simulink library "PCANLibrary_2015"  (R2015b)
settings: Solver=VariableStepAuto  SolverMode=SingleTasking  StartTime=0.0  StopTime=10.0  RelTol=1e-3
undefined symbols (not defined in the file or in its folder): FromID, hex2dec, Initvar, MsgFormat, PCAN_USBBUS, pcanchannel, ToID

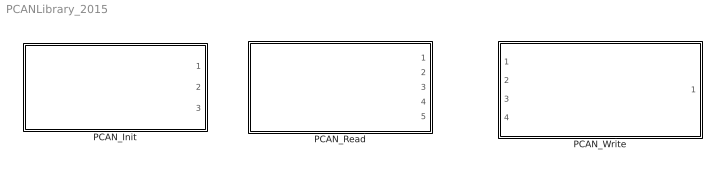
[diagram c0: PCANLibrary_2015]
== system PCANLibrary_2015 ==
  PCAN_Init : Subsystem
  PCAN_Read : Subsystem
  PCAN_Write : Subsystem

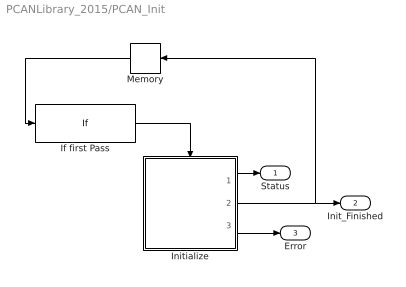
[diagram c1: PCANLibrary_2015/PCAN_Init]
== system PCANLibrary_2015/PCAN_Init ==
  If first Pass : If  IfExpression=u1 == 0  ShowElse=off
  Initialize : Subsystem  TreatAsAtomicUnit=on
  Memory : Memory  InheritSampleTime=on
  Status : Outport
  Init_Finished : Outport  Port=2
  Error : Outport  Port=3
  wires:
  If first Pass/1 -> Initialize/Action
  Initialize/1(Status) -> Status/1
  Memory/1 -> If first Pass/1
  Initialize/2(Init_Finished) -> Init_Finished/1, Memory/1
  Initialize/3(Error) -> Error/1

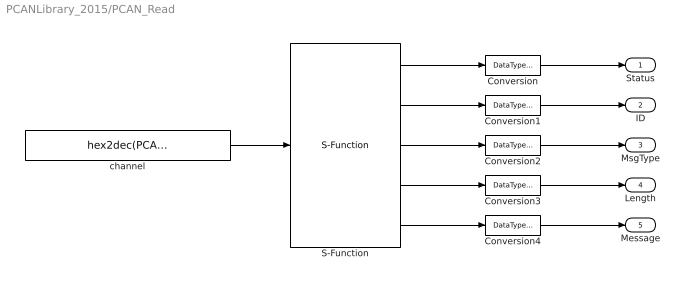
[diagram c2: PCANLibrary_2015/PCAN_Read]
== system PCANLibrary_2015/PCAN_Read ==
  Conversion : DataTypeConversion  OutDataTypeStr=uint32
  Conversion1 : DataTypeConversion  OutDataTypeStr=uint32
  Conversion2 : DataTypeConversion  OutDataTypeStr=uint8
  Conversion3 : DataTypeConversion  OutDataTypeStr=uint8
  Conversion4 : DataTypeConversion  OutDataTypeStr=uint8
  S-Function : S-Function  FunctionName=PCAN_Read  SFunctionDeploymentMode=off  EnableBusSupport=off
  channel : Constant  Value=hex2dec(PCAN_USBBUS)
  Status : Outport
  ID : Outport  Port=2
  MsgType : Outport  Port=3
  Length : Outport  Port=4
  Message : Outport  Port=5
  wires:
  S-Function/1 -> Conversion/1
  S-Function/2 -> Conversion1/1
  S-Function/3 -> Conversion2/1
  S-Function/4 -> Conversion3/1
  S-Function/5 -> Conversion4/1
  Conversion/1 -> Status/1
  Conversion1/1 -> ID/1
  Conversion2/1 -> MsgType/1
  Conversion3/1 -> Length/1
  Conversion4/1 -> Message/1
  channel/1 -> S-Function/1

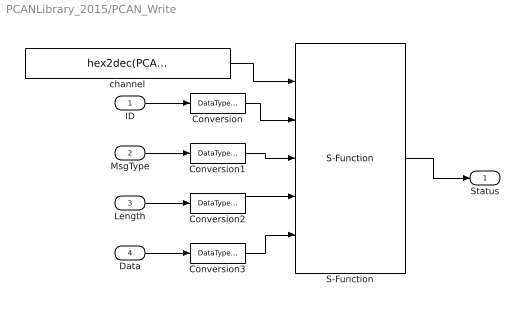
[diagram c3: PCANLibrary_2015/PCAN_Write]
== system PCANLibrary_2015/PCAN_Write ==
  ID : Inport  OutDataTypeStr=uint32
  MsgType : Inport  Port=2  OutDataTypeStr=uint8
  Length : Inport  Port=3  OutDataTypeStr=uint8
  Data : Inport  Port=4  OutDataTypeStr=uint8
  Conversion{,1..3} (4 alike) : DataTypeConversion  OutDataTypeStr=double
  S-Function : S-Function  FunctionName=PCAN_Write  SFunctionDeploymentMode=off  EnableBusSupport=off
  channel : Constant  Value=hex2dec(PCAN_USBBUS)
  Status : Outport
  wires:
  S-Function/1 -> Status/1
  ID/1 -> Conversion/1
  MsgType/1 -> Conversion1/1
  Length/1 -> Conversion2/1
  Data/1 -> Conversion3/1
  channel/1 -> S-Function/1
  Conversion/1 -> S-Function/2
  Conversion1/1 -> S-Function/3
  Conversion2/1 -> S-Function/4
  Conversion3/1 -> S-Function/5

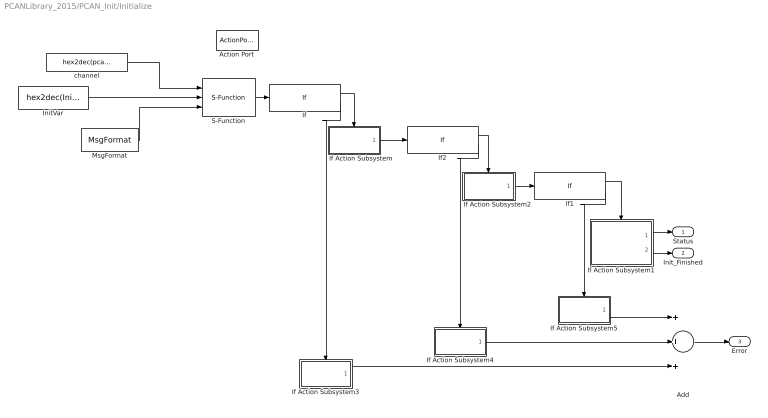
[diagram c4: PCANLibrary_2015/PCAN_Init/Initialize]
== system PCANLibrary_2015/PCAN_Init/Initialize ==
  Action Port : ActionPort
  Add : Sum  Inputs=+++
  If : If  IfExpression=u1== 0
  If Action Subsystem : Subsystem  TreatAsAtomicUnit=on
  If Action Subsystem1 : Subsystem  TreatAsAtomicUnit=on
  If Action Subsystem2 : Subsystem  TreatAsAtomicUnit=on
  If Action Subsystem3 : Subsystem  TreatAsAtomicUnit=on
  If Action Subsystem4 : Subsystem  TreatAsAtomicUnit=on
  If Action Subsystem5 : Subsystem  TreatAsAtomicUnit=on
  If1 : If  IfExpression=u1== 0
  If2 : If  IfExpression=u1== 0
  InitVar : Constant  Value=hex2dec(Initvar)
  MsgFormat : Constant  Value=MsgFormat
  S-Function : S-Function  FunctionName=PCAN_Init  SFunctionDeploymentMode=off  EnableBusSupport=off
  channel : Constant  Value=hex2dec(pcanchannel)
  Status : Outport  InitialOutput=0
  Init_Finished : Outport  Port=2  InitialOutput=0
  Error : Outport  Port=3  InitialOutput=0
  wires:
  S-Function/1 -> If/1
  If/1 -> If Action Subsystem/Action
  If Action Subsystem/1(Return) -> If2/1
  If Action Subsystem1/1(Status) -> Status/1
  If Action Subsystem1/2(Init_finish) -> Init_Finished/1
  If1/1 -> If Action Subsystem1/Action
  If2/1 -> If Action Subsystem2/Action
  If Action Subsystem2/1(return) -> If1/1
  If/2 -> If Action Subsystem3/Action
  If2/2 -> If Action Subsystem4/Action
  If1/2 -> If Action Subsystem5/Action
  If Action Subsystem5/1(Error) -> Add/1
  If Action Subsystem4/1(Error) -> Add/2
  If Action Subsystem3/1(Error) -> Add/3
  Add/1 -> Error/1
  MsgFormat/1 -> S-Function/3
  InitVar/1 -> S-Function/2
  channel/1 -> S-Function/1

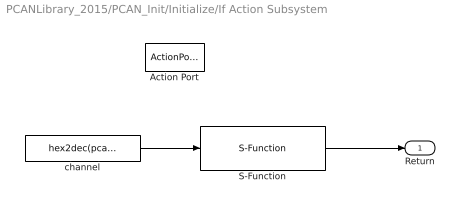
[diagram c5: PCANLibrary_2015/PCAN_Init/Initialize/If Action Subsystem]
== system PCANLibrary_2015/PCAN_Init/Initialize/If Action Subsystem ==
  Action Port : ActionPort
  S-Function : S-Function  FunctionName=PCAN_ResetFilter  SFunctionDeploymentMode=off  EnableBusSupport=off
  channel : Constant  Value=hex2dec(pcanchannel)
  Return : Outport
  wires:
  S-Function/1 -> Return/1
  channel/1 -> S-Function/1

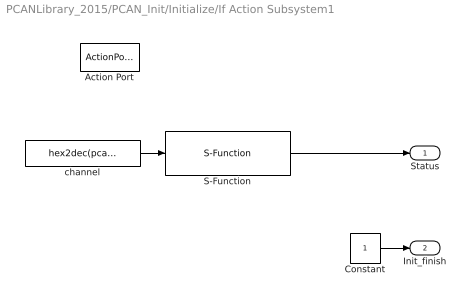
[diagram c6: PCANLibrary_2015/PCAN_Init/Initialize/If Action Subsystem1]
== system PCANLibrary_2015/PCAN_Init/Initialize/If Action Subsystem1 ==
  Action Port : ActionPort
  Constant : Constant
  S-Function : S-Function  FunctionName=PCAN_Status  SFunctionDeploymentMode=off  EnableBusSupport=off
  channel : Constant  Value=hex2dec(pcanchannel)
  Status : Outport
  Init_finish : Outport  Port=2
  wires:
  S-Function/1 -> Status/1
  Constant/1 -> Init_finish/1
  channel/1 -> S-Function/1

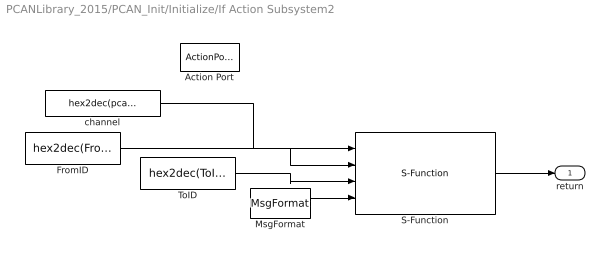
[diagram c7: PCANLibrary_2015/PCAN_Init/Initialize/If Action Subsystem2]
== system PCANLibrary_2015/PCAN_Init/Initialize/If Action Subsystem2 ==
  Action Port : ActionPort
  FromID : Constant  Value=hex2dec(FromID)
  MsgFormat : Constant  Value=MsgFormat
  S-Function : S-Function  FunctionName=PCAN_MsgFilter  SFunctionDeploymentMode=off  EnableBusSupport=off
  ToID : Constant  Value=hex2dec(ToID)
  channel : Constant  Value=hex2dec(pcanchannel)
  return : Outport
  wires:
  S-Function/1 -> return/1
  MsgFormat/1 -> S-Function/4
  ToID/1 -> S-Function/3
  FromID/1 -> S-Function/2
  channel/1 -> S-Function/1

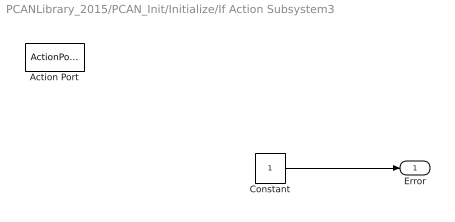
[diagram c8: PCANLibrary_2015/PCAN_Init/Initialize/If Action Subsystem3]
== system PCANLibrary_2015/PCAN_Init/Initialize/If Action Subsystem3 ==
  Action Port : ActionPort
  Constant : Constant
  Error : Outport  InitialOutput=0
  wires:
  Constant/1 -> Error/1

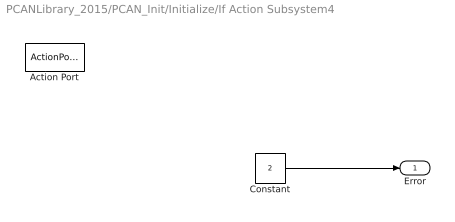
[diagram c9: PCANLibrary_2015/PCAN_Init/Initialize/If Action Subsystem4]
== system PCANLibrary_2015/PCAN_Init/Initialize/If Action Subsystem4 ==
  Action Port : ActionPort
  Constant : Constant  Value=2
  Error : Outport  InitialOutput=0
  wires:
  Constant/1 -> Error/1

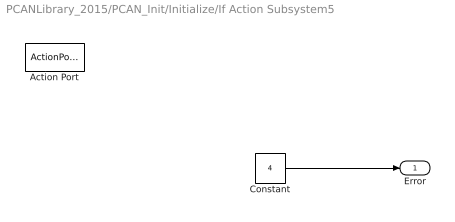
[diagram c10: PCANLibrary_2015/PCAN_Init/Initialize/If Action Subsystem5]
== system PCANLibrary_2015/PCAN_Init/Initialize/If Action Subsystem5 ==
  Action Port : ActionPort
  Constant : Constant  Value=4
  Error : Outport  InitialOutput=0
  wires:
  Constant/1 -> Error/1
